{attribute 'call_after_init'}
FUNCTION_BLOCK FB_DS_IED_LD1_LLN0_DS3 EXTENDS FB_AcsiCommonDataSetClass
VAR
END_VAR

METHOD OnInit : BOOL
VAR
END_VAR
IF NOT DeleteAllMembers() THEN RETURN; END_IF
IF NOT AddMember(ipData:=fbIED.IEDLD1.LEDGGIO1.ISCSO1, eFc:=E_AcsiFc.ST_) THEN RETURN; END_IF
IF NOT AddMember(ipData:=fbIED.IEDLD1.LEDGGIO2.ISCSO1, eFc:=E_AcsiFc.ST_) THEN RETURN; END_IF
IF NOT AddMember(ipData:=fbIED.IEDLD1.LEDGGIO3.ISCSO1, eFc:=E_AcsiFc.ST_) THEN RETURN; END_IF
IF NOT AddMember(ipData:=fbIED.IEDLD1.LEDGGIO4.ISCSO1, eFc:=E_AcsiFc.ST_) THEN RETURN; END_IF
IF NOT AddMember(ipData:=fbIED.IEDLD1.LEDGGIO5.ISCSO1, eFc:=E_AcsiFc.ST_) THEN RETURN; END_IF
IF NOT AddMember(ipData:=fbIED.IEDLD1.LEDGGIO6.ISCSO1, eFc:=E_AcsiFc.ST_) THEN RETURN; END_IF
IF NOT AddMember(ipData:=fbIED.IEDLD1.LEDGGIO7.ISCSO1, eFc:=E_AcsiFc.ST_) THEN RETURN; END_IF
IF NOT AddMember(ipData:=fbIED.IEDLD1.LEDGGIO8.ISCSO1, eFc:=E_AcsiFc.ST_) THEN RETURN; END_IF
OnInit:= TRUE;
END_METHOD

END_FUNCTION_BLOCK
